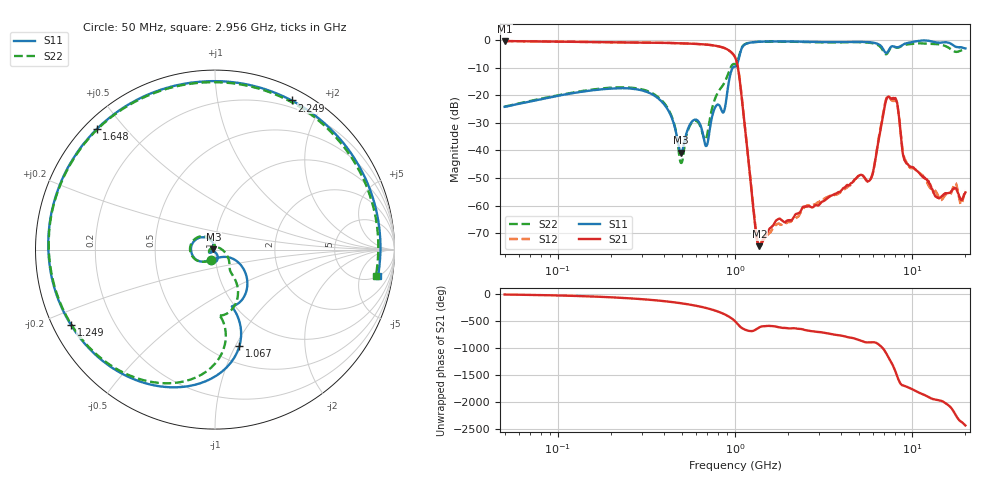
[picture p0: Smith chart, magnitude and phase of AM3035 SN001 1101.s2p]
# Hz S DB R 50
!freq MagS11 AngS11 MagS21 AngS21 MagS12 AngS12 MagS22 AngS22
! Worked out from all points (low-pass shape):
!   1601 points, 50 MHz to 20.05 GHz, reference 50 ohm
!   highest |S21| = -0.39 dB at 50 MHz (marker M1); lowest = -74.6 dB at 1.377 GHz (marker M2)
!   |S21| within 3 dB of the highest: start of sweep to 904.1 MHz
!   lowest |S11| = -40.8 dB at 496.9 MHz (marker M3), VSWR 1.02, Z = 49.1 + j0.143 ohm
!   |S11| at or under -10 dB: start of sweep to 972.5 MHz
!   |S22| runs from -44.5 to -0.6 dB; largest |S21 - S12| = 0.012
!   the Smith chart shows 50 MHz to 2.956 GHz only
!   S11 on the Smith chart (normalised r, x): 50 MHz: 0.95, -0.11; 1.067 GHz: 0.67, -1.04; 1.249 GHz: 0.05, -0.24; 1.648 GHz: 0.04, +0.42; 2.249 GHz: 0.12, +1.63; 2.956 GHz: 5, -10
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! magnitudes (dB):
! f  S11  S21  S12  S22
! 50 MHz  -24.2  -0.4  -0.4  -24.1
! 135.9 MHz  -18.7  -0.7  -0.7  -18.5
! 369.6 MHz  -21.2  -1.0  -1.0  -20.8
! 440.8 MHz  -28.3  -1.1  -1.1  -27.9
! 496.9 MHz  -40.8  -1.2  -1.2  -44.5
! 590.4 MHz  -28.9  -1.4  -1.4  -29.2
! 693.6 MHz  -38.2  -1.7  -1.7  -34.9
! 1.005 GHz  -9.6  -6.4  -6.4  -8.8
! 1.067 GHz  -5.1  -15.1  -14.7  -4.7
! 1.249 GHz  -0.9  -56.2  -55.7  -0.8
! 1.377 GHz  -0.6  -74.6  -74.2  -0.6
! 1.648 GHz  -0.5  -67.0  -68.2  -0.6
! 2.249 GHz  -0.6  -62.8  -64.1  -0.7
! 2.722 GHz  -0.7  -60.6  -59.9  -0.8
! 2.956 GHz  -0.7  -59.9  -58.7  -0.8
! 5.802 GHz  -0.8  -50.7  -50.8  -1.0
! 7.402 GHz  -3.7  -20.5  -20.6  -4.0
! 8.159 GHz  -2.6  -21.8  -22.5  -2.8
! 8.96 GHz  -1.6  -42.3  -41.7  -1.8
! 9.585 GHz  -1.0  -45.4  -45.6  -1.6
! 14.53 GHz  -1.0  -57.0  -57.9  -1.7
! 20.05 GHz  -3.1  -55.2  -54.2  -3.6
